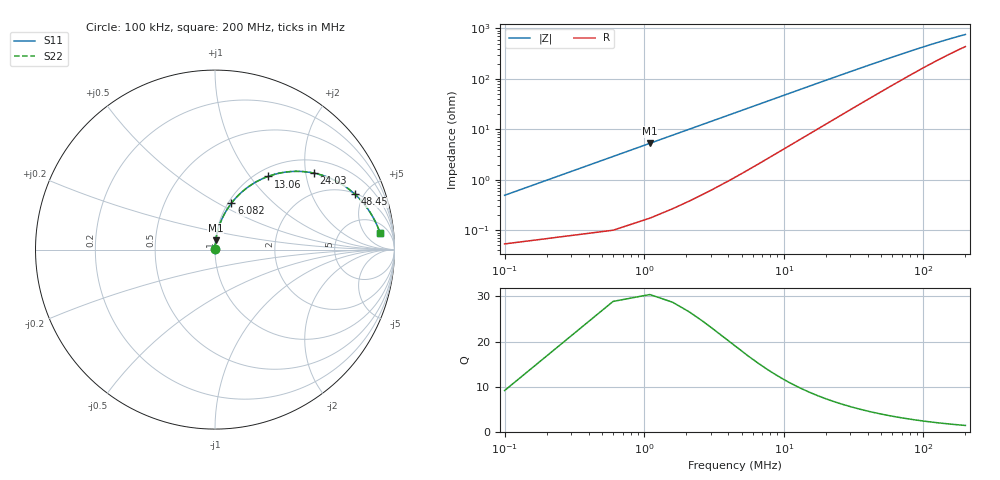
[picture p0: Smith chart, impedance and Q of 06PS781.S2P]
! Coilcraft 0603PS-781 Power Chip Inductor
! 19 February 2003
# MHZ S MA R 50
!Freq  MagS11  AngS11  MagS21  AngS21  MagS12  AngS12  MagS22  AngS22
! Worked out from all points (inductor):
!   403 points, 100 kHz to 200 MHz, reference 50 ohm
!   read as one part in series: L = 763 nH near 1.097 MHz
!   highest Q = 24.6 at 1.097 MHz (marker M1), where L = 765 nH
!   S11 on the Smith chart (normalised r, x): 100 kHz: 1.00, +0.01; 6.082 MHz: 1.04, +0.58; 13.06 MHz: 1.13, +1.23; 24.03 MHz: 1.34, +2.22; 48.45 MHz: 2.07, +4.30; 200 MHz: 10, +12
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0.1  0.004928 83.5  0.9995 -0.3  0.9995 -0.3  0.004928 83.5
0.5985  0.02888 86.4  0.9986 -1.7  0.9986 -1.7  0.02888 86.4
1.097  0.05258 85.1  0.9969 -3.0  0.9969 -3.0  0.05258 85.1
1.5955  0.07607 83.6  0.9945 -4.4  0.9945 -4.4  0.07607 83.6
2.094  0.09934 82.2  0.9913 -5.7  0.9913 -5.7  0.09934 82.2
2.5925  0.1224 80.7  0.9875 -7.0  0.9875 -7.0  0.1224 80.7
3.091  0.1451 79.2  0.9831 -8.3  0.9831 -8.3  0.1451 79.2
4.088  0.1895 76.2  0.9724 -10.9  0.9724 -10.9  0.1895 76.2
6.082  0.2735 70.6  0.9449 -15.8  0.9449 -15.8  0.2735 70.6
7.5775  0.3314 66.6  0.92 -19.3  0.92 -19.3  0.3314 66.6
9.073  0.3845 62.8  0.8927 -22.5  0.8927 -22.5  0.3845 62.8
13.061  0.503 54.1  0.8144 -30.0  0.8144 -30.0  0.503 54.1
18.046  0.6105 45.5  0.7187 -37.3  0.7187 -37.3  0.6105 45.5
24.028  0.6964 37.7  0.6193 -43.5  0.6193 -43.5  0.6964 37.7
33.4995  0.7766 29.4  0.4999 -49.7  0.4999 -49.7  0.7766 29.4
40.4785  0.8117 25.2  0.4354 -52.5  0.4354 -52.5  0.8117 25.2
48.4545  0.8386 21.6  0.3788 -54.5  0.3788 -54.5  0.8386 21.6
66.899  0.8738 16.2  0.2914 -56.5  0.2914 -56.5  0.8738 16.2
100.2985  0.9012 11.1  0.2081 -56.3  0.2081 -56.3  0.9012 11.1
133.698  0.9135 8.4  0.1648 -54.2  0.1648 -54.2  0.9135 8.4
167.0975  0.9205 6.8  0.1387 -51.7  0.1387 -51.7  0.9205 6.8
200  0.9251 5.7  0.1216 -49.2  0.1216 -49.2  0.9251 5.7
